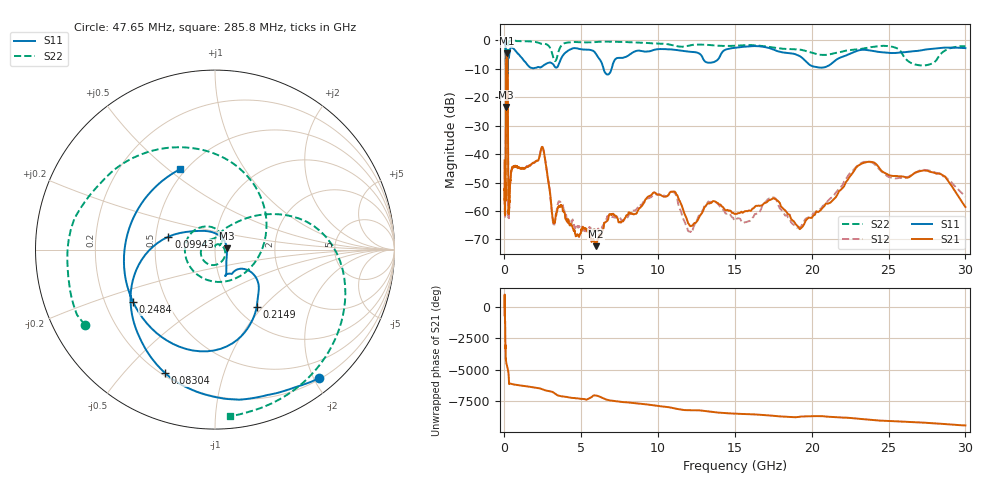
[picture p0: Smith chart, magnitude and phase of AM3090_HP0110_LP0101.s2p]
! Date/Time: Thu, Feb 28, 2019 1:59 PM
! Network Analyzer: Agilent Technologies E8364B Rev: A.07.50.67
! Sweep from 0.010 to 30.000 GHz, 1601 Points, Sweep Type: LOG
! Power Supply: 5.023 V, 0.002 A
# Hz S DB R 50
!freq MagS11 AngS11 MagS21 AngS21 MagS12 AngS12 MagS22 AngS22
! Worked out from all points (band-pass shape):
!   1601 points, 10 MHz to 30 GHz, reference 50 ohm
!   highest |S21| = -4.65 dB at 152.1 MHz (marker M1); lowest = -72.3 dB at 5.959 GHz (marker M2)
!   |S21| within 3 dB of the highest: 110.3 MHz to 202.5 MHz (92.2 MHz wide, 59 % of centre)
!   lowest |S11| = -23.5 dB at 107.7 MHz (marker M3), VSWR 1.14, Z = 57.1 + j0.847 ohm
!   |S11| at or under -10 dB: 98.52 MHz to 203.6 MHz (105.1 MHz wide, 69.6 % of centre); 6.447 GHz to 6.978 GHz (531.3 MHz wide, 7.92 % of centre)
!   |S22| runs from -35.2 to -0.1 dB; largest |S21 - S12| = 0.015
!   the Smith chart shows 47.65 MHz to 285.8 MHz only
!   S11 on the Smith chart (normalised r, x): 47.65 MHz: 0.23, -2.07; 83.04 MHz: 0.21, -0.65; 99.43 MHz: 0.58, +0.09; 214.9 MHz: 1.22, -0.93; 248.4 MHz: 0.32, -0.27; 285.8 MHz: 0.47, +0.55
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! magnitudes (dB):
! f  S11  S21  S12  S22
! 10 MHz  -0.3  -42.2  -42.8  -0.6
! 38.04 MHz  -0.5  -59.5  -59.9  -1.4
! 47.65 MHz  -0.7  -50.8  -50.7  -1.5
! 83.04 MHz  -2.6  -49.8  -51.1  -5.3
! 99.43 MHz  -11.4  -16.7  -16.7  -15.2
! 107.7 MHz  -23.5  -8.6  -8.6  -16.0
! 131.6 MHz  -16.1  -5.0  -5.0  -34.9
! 144.7 MHz  -16.4  -4.7  -4.7  -27.2
! 152.1 MHz  -16.2  -4.6  -4.6  -23.9
! 214.9 MHz  -8.0  -12.9  -12.8  -11.3
! 248.4 MHz  -5.3  -56.0  -58.6  -1.4
! 285.8 MHz  -6.2  -59.8  -61.2  -0.6
! 550.5 MHz  -2.9  -44.4  -44.6  -0.2
! 2.084 GHz  -9.7  -42.4  -42.5  -0.7
! 2.533 GHz  -8.9  -38.4  -38.4  -1.3
! 3.22 GHz  -8.9  -64.1  -64.9  -6.9
! 5.959 GHz  -4.9  -72.3  -67.1  -0.7
! 7.926 GHz  -5.9  -61.6  -62.6  -0.7
! 10.7 GHz  -3.3  -54.1  -54.3  -1.5
! 19.41 GHz  -6.4  -65.4  -64.2  -3.6
! 23.59 GHz  -3.5  -42.8  -42.7  -2.7
! 30 GHz  -2.8  -58.6  -55.0  -2.2
